(* Logix 5000 Rung export; software revision 20.03 *)

TYPE PSILX56DPMasterControl :
STRUCT
   ControlCommand : SINT;   // 0 - Profibus OFFLINE 1 - Profibus STOPPED 2 - Profibus CLEAR 3 - Profibus OPERATIONAL
   RedundancyControl : SINT;
   Reserved : INT;
   DeviceEnable : BOOL[128];
END_STRUCT
END_TYPE

TYPE PSILX56DPMasterStatus :
STRUCT
   ConfigValid : BOOL;
   Owned : BOOL;
   DuplicateDPStation : BOOL;
   ProfibusFieldbusError : BOOL;
   ProfibusDeviceError : BOOL;
   ProfibusOffline : BOOL;
   ProfibusStopped : BOOL;
   ProfibusClear : BOOL;
   ProfibusOperational : BOOL;
   SlaveMode : BOOL;
   Reserved0 : INT;
   ConfigCRC : INT;
   ActiveNodeCount : SINT;
   Reserved : SINT;
   SwitchOverTimeout : INT;
   Reserved2 : INT;
   DeviceLiveList : BOOL[128];
   DeviceDataExchangeActive : BOOL[128];
   DeviceAlarmPendingFlags : BOOL[128];
   DeviceDiagnosticPendingFlags : BOOL[128];
END_STRUCT
END_TYPE

VAR_GLOBAL   (* controller tags *)
   Local:6:O : AB:1756_MODULE_SINT_496Bytes:O:0;
   ILX56PBM_MasterStatus : PSILX56DPMasterStatus;
   ILX56PBM_MasterControl : PSILX56DPMasterControl := (ControlCommand := 3, DeviceEnable[2] := 1, DeviceEnable[3] := 1, DeviceEnable[12] := 1, DeviceEnable[13] := 1, DeviceEnable[22] := 1, DeviceEnable[23] := 1);
   Local:6:I : AB:1756_MODULE_SINT_500Bytes:I:0;
END_VAR

PROGRAM MainProgram

ROUTINE ILX56_PBM1Map   (* ladder *)
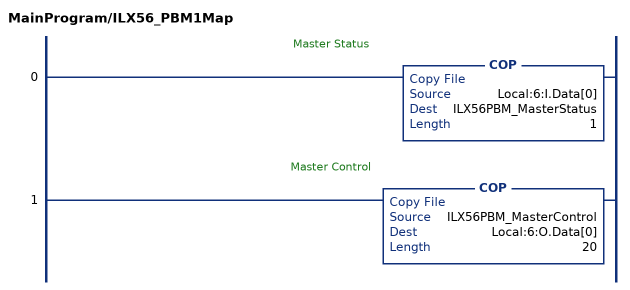
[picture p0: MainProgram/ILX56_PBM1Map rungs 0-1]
   // Master Status
   0: COP(Local:6:I.Data[0],ILX56PBM_MasterStatus,1);
   // Master Control
   1: COP(ILX56PBM_MasterControl,Local:6:O.Data[0],20);
END_ROUTINE
END_PROGRAM
